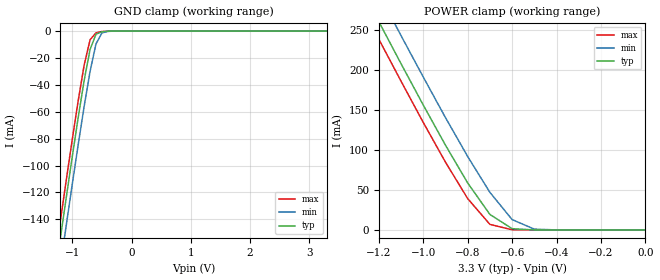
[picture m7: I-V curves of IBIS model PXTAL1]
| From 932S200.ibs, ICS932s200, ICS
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|   Model PXTAL1
[Model]   PXTAL1
Model_type   Input
Polarity   Non-Inverting
Vinl = 800.00mV
Vinh =   2.00V
C_comp   5.50pF   5.00pF   6.00pF
[Temperature Range]   27.00   70.00   0.00
[Voltage Range]   3.30V   3.00V   3.70V
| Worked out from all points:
|   GND clamp passes 1 mA (typ) near -0.53 V on its own axis
|   POWER clamp passes 1 mA (typ) near -0.56 V on its own axis
[GND_clamp]
| voltage   I(typ)   I(min)   I(max)
-3.3V     -818.7mA   -838.4mA   -806.5mA
-1.3V     -184.4mA   -205.1mA   -171.6mA
-1.2V     -153.6mA   -174.3mA   -140.8mA
-1.1V     -123.2mA   -143.8mA   -110.3mA
-1V       -93.23mA   -113.8mA   -80.48mA
-900mV    -64.14mA   -84.35mA   -51.7mA
-800mV    -36.72mA   -56.02mA   -25.33mA
-700mV    -13.63mA   -29.93mA   -6.41mA
-600mV    -2.31mA    -9.53mA    -1.31mA
-500mV    -487.9uA   -1.36mA    -326.3uA
-400mV    -91uA      -228.6uA   -44.4uA
3.3V      108.9pA    1.5uA      48.42pA
[POWER_clamp]
| voltage   I(typ)   I(min)   I(max)
-3.3V     1.41A      1.44A      1.39A
-1.3V     314.3mA    349.5mA    292.4mA
-1.2V     261.1mA    296.3mA    239.1mA
-1.1V     208.4mA    243.6mA    186.5mA
-1V       156.6mA    191.7mA    134.8mA
-900mV    106.3mA    140.8mA    85.01mA
-800mV    58.94mA    92.02mA    39.34mA
-700mV    19.46mA    47.14mA    7mA
-600mV    1.61mA     13.03mA    241.9uA
-500mV    48.08uA    1.03mA     4.48uA
-400mV    1.09uA     42.41uA    71.42nA
0V        108.9pA    1.22nA     66.46pA
